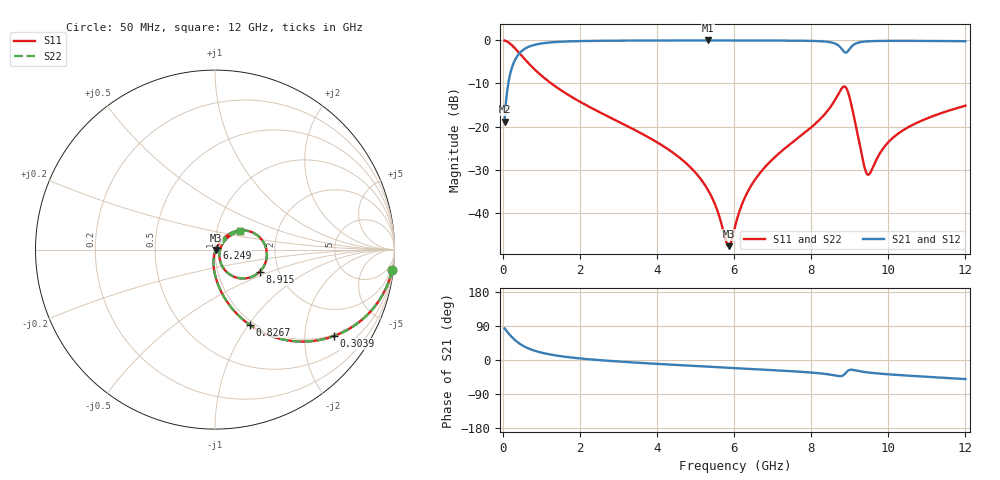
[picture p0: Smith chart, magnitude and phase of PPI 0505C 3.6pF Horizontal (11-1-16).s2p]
# MHz S MA R 50
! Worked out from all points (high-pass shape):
!   1601 points, 50 MHz to 12 GHz, reference 50 ohm
!   highest |S21| = -0.04 dB at 5.315 GHz (marker M1); lowest = -18.9 dB at 50 MHz (marker M2)
!   |S21| within 3 dB of the highest: 432.1 MHz to end of sweep
!   lowest |S11| = -47.7 dB at 5.861 GHz (marker M3), VSWR 1.01, Z = 50.4 - j0.148 ohm
!   |S11| at or under -10 dB: 1.261 GHz to end of sweep
!   |S22| runs from -47.7 to -0.1 dB; largest |S21 - S12| = 0
!   S11 on the Smith chart (normalised r, x): 50 MHz: 1, -17; 303.9 MHz: 0.95, -2.79; 826.8 MHz: 0.95, -1.01; 6.249 GHz: 1.02, +0.02; 8.915 GHz: 1.59, -0.43; 12 GHz: 1.29, +0.28
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50  0.9935 -6.7  0.1139 83.3  0.1139 83.3  0.9935 -6.7
169.5  0.9318 -21.9  0.3625 68.1  0.3625 68.1  0.9318 -21.9
303.9375  0.8195 -36.0  0.5724 54.0  0.5724 54.0  0.8195 -36.0
550.4062  0.6179 -53.7  0.7851 36.2  0.7851 36.2  0.6179 -53.7
826.75  0.4605 -65.3  0.8862 24.5  0.8862 24.5  0.4605 -65.3
2044.156  0.1898 -85.5  0.9794 3.8  0.9794 3.8  0.1898 -85.5
4038.312  0.06443 -97.6  0.9945 -10.4  0.9945 -10.4  0.06443 -97.6
4807.594  0.03587 -99.1  0.9955 -14.7  0.9955 -14.7  0.03587 -99.1
5315.469  0.01873 -95.8  0.9957 -17.4  0.9957 -17.4  0.01873 -95.8
5860.688  0.004118 -20.9  0.9955 -20.3  0.9955 -20.3  0.004118 -20.9
6025  0.006972 31.4  0.9954 -21.2  0.9954 -21.2  0.006972 31.4
6249.062  0.01399 49.2  0.9951 -22.4  0.9951 -22.4  0.01399 49.2
6839.094  0.03539 56.1  0.9938 -25.6  0.9938 -25.6  0.03539 56.1
8019.156  0.09967 50.3  0.9833 -33.2  0.9833 -33.2  0.09967 50.3
8661.469  0.2202 27.2  0.8981 -41.5  0.8981 -41.5  0.2202 27.2
8915.406  0.2774 -26.5  0.723 -32.0  0.723 -32.0  0.2774 -26.5
9124.531  0.1215 -64.9  0.9009 -26.9  0.9009 -26.9  0.1215 -64.9
9356.062  0.03798 -49.8  0.9634 -31.2  0.9634 -31.2  0.03798 -49.8
9453.156  0.02805 -20.4  0.972 -32.6  0.972 -32.6  0.02805 -20.4
10013.31  0.06686 41.7  0.985 -37.8  0.985 -37.8  0.06686 41.7
10745.25  0.1109 42.7  0.9843 -42.7  0.9843 -42.7  0.1109 42.7
12000  0.1748 36.9  0.9757 -50.4  0.9757 -50.4  0.1748 36.9
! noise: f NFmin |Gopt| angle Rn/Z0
50  0.0006471  0.9265  1.846  0.001951
1372  0.005208  0.7412  5.607  0.004025
2701  0.008441  0.6946  9.981  0.005353
4031  0.01139  0.6691  14.38  0.006514
5360  0.01438  0.6565  18.72  0.007784
6682  0.01811  0.662  22.96  0.009865
8012  0.02967  0.7433  27.28  0.02194
9341  0.0588  0.8423  31.9  0.07318
1.067e+04  0.03064  0.6878  35.71  0.01733
1.2e+04  0.03096  0.663  39.45  0.01567
